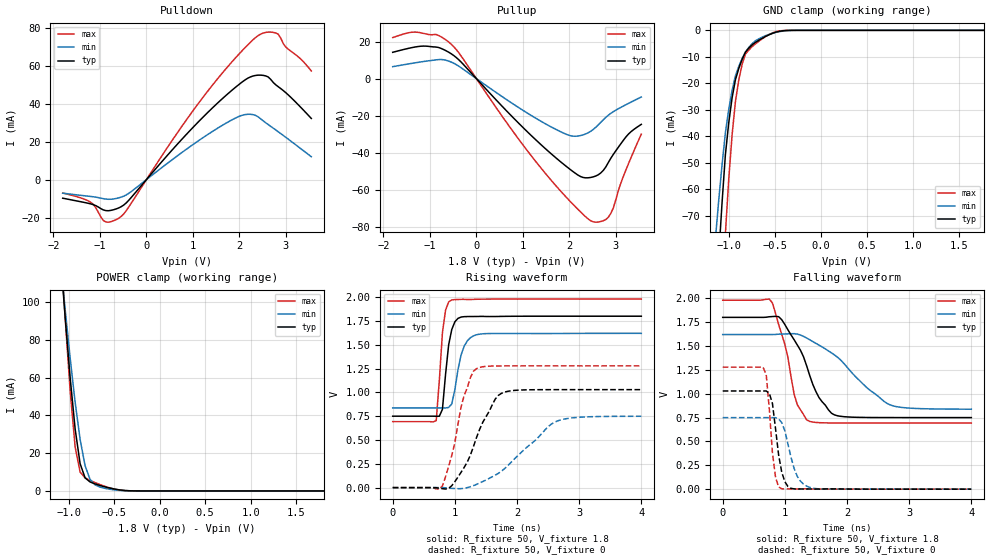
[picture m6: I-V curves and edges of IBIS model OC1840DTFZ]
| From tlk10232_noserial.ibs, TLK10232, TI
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[Model]   OC1840DTFZ
Model_type   3-state
Polarity   Non-Inverting
Enable   Active-Low
Cref =  15.0000pF
Rref =  100.0000M
Vref =  0V
Vmeas =  0.9
C_comp   1.176081p   0.9499518p   1.481389p
[Temperature Range]   25   125   -40
[Voltage Range]   1.8   1.62   1.98
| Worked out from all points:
|   slope of the pulldown table from 0 to 0.27 V, typ, clamps not added: 34.9 ohm
|   slope of the pullup table from 0 to 0.27 V, typ, clamps not added: 36.8 ohm
|   GND clamp passes 1 mA (typ) near -0.52 V on its own axis
|   POWER clamp passes 1 mA (typ) near -0.50 V on its own axis
|   rising waveform, R_fixture 50, V_fixture 1.8: 20-80 % time 109ps typ, 149ps min, 90.8ps max; typ from 0.75 V to 1.8 V
|   rising waveform, R_fixture 50, V_fixture 0: 20-80 % time 425ps typ, 742ps min, 270ps max; typ from 0 V to 1.03 V
|   falling waveform, R_fixture 50, V_fixture 1.8: 20-80 % time 424ps typ, 795ps min, 268ps max; typ from 1.8 V to 0.75 V
|   falling waveform, R_fixture 50, V_fixture 0: 20-80 % time 128ps typ, 186ps min, 99.8ps max; typ from 1.03 V to 0 V
[POWER_clamp]
-1.8V     632.5mA    513.6mA    762.8mA
-1.055V   103.2mA    104.9mA    105.7mA
-1.036V   91.74mA    95.93mA    91.47mA
-981.8mV  59.9mA     70.34mA    52.88mA
-927.3mV  32.78mA    46.98mA    23.28mA
-872.7mV  14.44mA    27.29mA    9.984mA
-818.2mV  6.921mA    13.34mA    6.938mA
-763.6mV  4.752mA    6.081mA    5.583mA
-709.1mV  3.714mA    3.231mA    4.428mA
-654.5mV  2.886mA    2.042mA    3.366mA
-381.8mV  235.3uA    109.3uA    182.9uA
1.8V      215.7nA    182nA      306.8nA
[Pulldown]
-1.8V     -9.787mA   -7.157mA   -7.07mA
-1.2V     -12.77mA   -8.858mA   -11.91mA
-872.7mV  -16.33mA   -10.26mA   -22.33mA
-545.5mV  -14.3mA    -9.25mA    -19.44mA
872.7mV   24.19mA    16.25mA    31.94mA
1.745V    45.14mA    30.24mA    59.46mA
2.127V    52.67mA    34.31mA    69.73mA
2.455V    55.09mA    32.1mA     76.69mA
2.618V    54.12mA    29.03mA    77.78mA
2.836V    48.95mA    25.2mA     76.64mA
3V        45.75mA    22.24mA    69.85mA
3.545V    32.26mA    12.07mA    57.29mA
[Pullup]
-1.8V     14.19mA    6.456mA    22.11mA
-1.255V   17.3mA     8.779mA    24.95mA
-872.7mV  17.03mA    10.1mA     23.81mA
-545.5mV  13.45mA    8.957mA    18.63mA
927.3mV   -24.47mA   -15.88mA   -33.23mA
1.8V      -44.56mA   -28.46mA   -60.23mA
2.127V    -50.96mA   -31.02mA   -68.97mA
2.509V    -52.9mA    -27.4mA    -77.08mA
2.727V    -49.43mA   -22.16mA   -76.51mA
2.891V    -42.81mA   -18.65mA   -72.53mA
3.273V    -29.75mA   -13.28mA   -45.61mA
3.545V    -24.61mA   -9.874mA   -29.89mA
[GND_clamp]
-1.8V     -615.2mA   -425.7mA   -961.8mA
-1.145V   -108mA     -79.2mA    -177.9mA
-1.109V   -85.62mA   -64.44mA   -141.2mA
-1.073V   -65.28mA   -50.94mA   -107.5mA
-1.036V   -47.02mA   -38.71mA   -76.91mA
-963.6mV  -25.46mA   -22.7mA    -39.54mA
-927.3mV  -18.64mA   -17.14mA   -26.82mA
-890.9mV  -14.38mA   -13.6mA    -18.72mA
-818.2mV  -8.226mA   -8.111mA   -8.937mA
-709.1mV  -4.493mA   -3.908mA   -5.066mA
-418.2mV  -195.3uA   -310.3uA   -95.1uA
1.764V    196.1nA    921nA      196.2nA
[Ramp]
dV/dt_f  0.6369169/0.4308171n   0.474941/0.8095593n  0.7794575/0.2680672n
dV/dt_r  0.6262443/0.4351261n  0.4563956/0.7617344n  0.7769396/0.2744914n
R_load = 50
[Rising Waveform]
R_fixture = 50
V_fixture = 1.8
V_fixture_min = 1.62
V_fixture_max = 1.98
0s        749.9mV    837.3mV    692.7mV
700ps     749.5mV    837.3mV    702.8mV
800ps     821.9mV    837.7mV    1.627V
850ps     1.187V     836.2mV    1.863V
900ps     1.498V     842mV      1.95V
950ps     1.66V      878.4mV    1.971V
1.1ns     1.791V     1.393V     1.977V
1.2ns     1.796V     1.54V      1.976V
1.3ns     1.797V     1.594V     1.977V
4ns       1.8V       1.62V      1.98V
[Rising Waveform]
R_fixture = 50
V_fixture = 0
V_fixture_min = 0
V_fixture_max = 0
0s        629.3nV    577.8nV    735.1nV
800ps     -11.34mV   391.7uV    16.98mV
950ps     20.02mV    -7.893mV   335.9mV
1.15ns    212.5mV    -7.267mV   968.4mV
1.25ns    341.7mV    9.173mV    1.156V
1.35ns    528.9mV    34.2mV     1.25V
1.65ns    930.1mV    130.7mV    1.277V
1.8ns     1.003V     199.3mV    1.278V
2.65ns    1.029V     699.8mV    1.278V
4ns       1.029V     749.1mV    1.278V
[Falling Waveform]
R_fixture = 50
V_fixture = 1.8
V_fixture_min = 1.62
V_fixture_max = 1.98
0s        1.8V       1.62V      1.98V
800ps     1.809V     1.62V      1.951V
1ns       1.725V     1.626V     1.517V
1.15ns    1.565V     1.629V     992mV
1.2ns     1.511V     1.625V     885.3mV
1.4ns     1.191V     1.565V     709.7mV
1.55ns    959.2mV    1.509V     696.9mV
1.85ns    768.5mV    1.381V     693.1mV
2.7ns     750.2mV    881.6mV    692.7mV
4ns       749.9mV    837.9mV    692.7mV
[Falling Waveform]
R_fixture = 50
V_fixture = 0
V_fixture_min = 0
V_fixture_max = 0
0s        1.029V     749.3mV    1.278V
650ps     1.028V     749.3mV    1.276V
700ps     1.029V     749.3mV    1.2V
800ps     898.4mV    749.7mV    380.5mV
850ps     633.9mV    749.3mV    124.8mV
950ps     177.7mV    696.8mV    3.955mV
1.05ns    27.33mV    471.6mV    2.884mV
1.2ns     2.017mV    134mV      1.512mV
1.4ns     1.958mV    18.6mV     3.241mV
4ns       690.2nV    79.44uV    735.8nV
